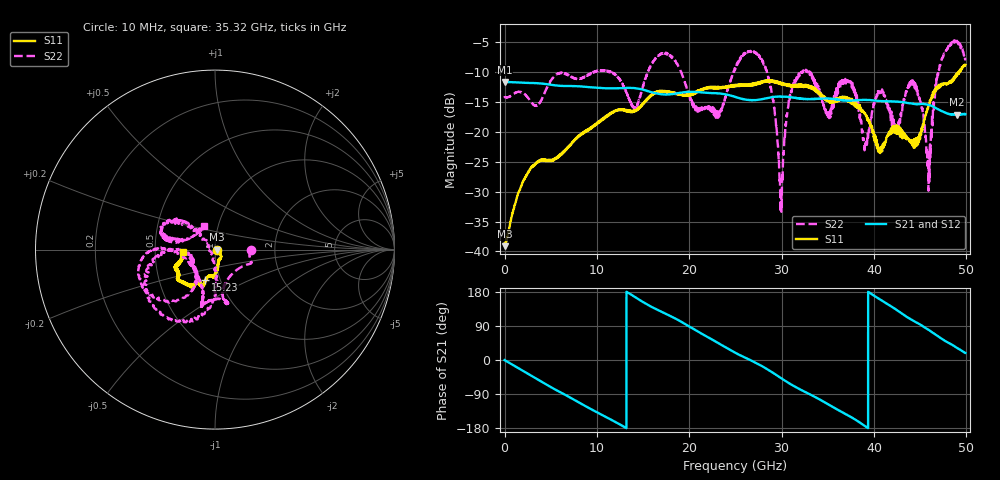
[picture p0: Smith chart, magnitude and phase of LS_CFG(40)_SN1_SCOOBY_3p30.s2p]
!Keysight Technologies,N5245B,MY58422026,A.13.80.08
!Date: Thursday, March 19, 2020 23:39:22
!Correction: S11(Full 2 Port(1,2))
!S21(Full 2 Port(1,2))
!S12(Full 2 Port(1,2))
!S22(Full 2 Port(1,2))
!S2P File: Measurements: S11, S21, S12, S22:
# Hz S DB R 50.0
!freq dBS11 angS11 dBS21 angS21 dBS12 angS12 dBS22 angS22
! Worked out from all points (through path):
!   4991 points, 10 MHz to 49.91 GHz, reference 50 ohm
!   highest |S21| = -11.69 dB at 20 MHz (marker M1); lowest = -17.2 dB at 49 GHz (marker M2)
!   group delay of S21, straight-line fit = 38.5 ps
!   lowest |S11| = -39.1 dB at 20 MHz (marker M3), VSWR 1.02, Z = 51.1 - j0.0956 ohm
!   |S11| at or under -10 dB: start of sweep to 49.24 GHz; 49.29918 GHz to 49.33088 GHz (31.71 MHz wide, 0.0643 % of centre)
!   |S22| runs from -33.4 to -4.8 dB; largest |S21 - S12| = 0.0025
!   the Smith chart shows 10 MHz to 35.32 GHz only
!   S11 on the Smith chart (normalised r, x): 10 MHz: 1.02, -0.01; 15.23 GHz: 0.85, -0.30; 35.32 GHz: 0.70, -0.02
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1e7  -38.67 -14.2  -11.70 -0.3  -11.69 -0.3  -14.06 -0.1
2e7  -39.11 -4.8  -11.69 -0.4  -11.69 -0.4  -14.19 -0.5
2.76e9  -26.33 -45.5  -11.87 -39.3  -11.86 -39.2  -14.79 -30.2
8.33e9  -20.52 -80.9  -12.45 -115.8  -12.45 -115.7  -11.09 -92.4
1.523e10  -14.90 -107.9  -13.10 149.5  -13.09 149.6  -11.14 178.9
1.665e10  -13.35 -108.7  -13.68 131.2  -13.68 131.2  -7.33 -167.9
2.3e10  -12.78 -120.6  -13.59 46.8  -13.59 46.9  -17.48 -156.9
2.496e10  -12.37 -124.7  -14.17 19.5  -14.16 19.6  -9.56 -170.7
2.818e10  -11.69 -138.6  -14.48 -20.3  -14.48 -20.2  -9.10 -99.3
2.992e10  -11.86 -144.6  -14.16 -47.6  -14.16 -47.4  -30.69 -165.1
3.112e10  -12.27 -149.5  -14.29 -65.7  -14.31 -65.4  -12.83 135.8
3.328e10  -12.62 -159.0  -14.54 -93.4  -14.54 -93.0  -10.67 167.6
3.532e10  -14.94 -175.4  -14.49 -120.6  -14.43 -120.2  -16.46 115.7
3.735e10  -14.91 171.5  -14.80 -148.4  -14.72 -148.5  -11.68 128.0
3.904e10  -16.92 174.2  -14.68 -174.4  -14.67 -174.6  -22.77 -121.6
4.044e10  -23.00 155.0  -14.86 163.2  -14.86 163.1  -13.31 -10.9
4.16e10  -20.17 102.7  -14.94 145.9  -14.96 145.8  -16.25 16.5
4.436e10  -21.27 57.9  -15.37 102.1  -15.40 102.1  -11.90 -24.4
4.591e10  -15.62 3.7  -15.51 79.8  -15.53 79.8  -29.85 -62.6
4.711e10  -12.16 7.5  -16.39 60.0  -16.40 60.1  -9.06 -100.9
4.9e10  -10.42 -16.3  -17.17 32.0  -17.18 32.1  -4.83 -48.4
4.991e10  -8.87 -16.1  -17.07 18.5  -17.09 18.4  -7.88 -23.1
